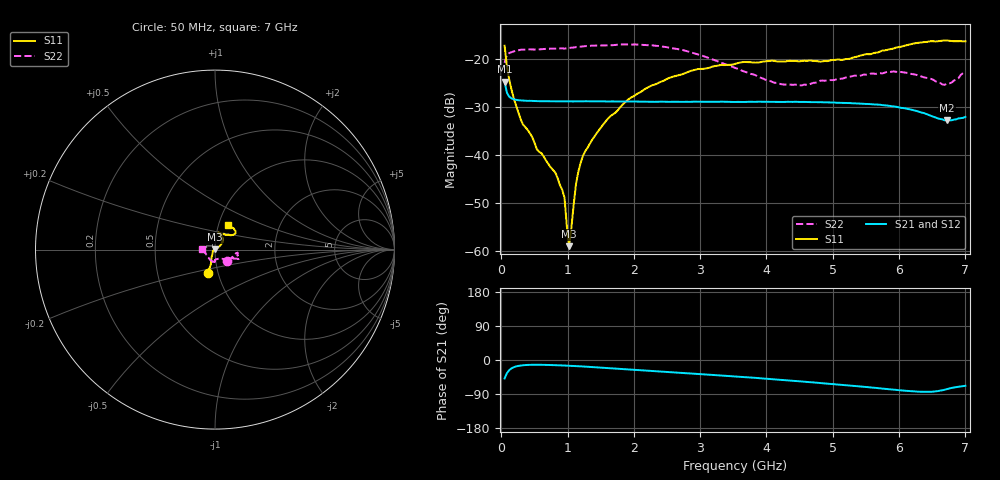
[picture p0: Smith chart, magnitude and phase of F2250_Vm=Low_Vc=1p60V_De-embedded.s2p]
! Integrated Device Technology
! Corporate Headquarters
! 6024 Silver Creek Valley Road
! San Jose, CA 95138  USA
! Phone:  1-408-284-8200
! Toll Free:  1-800-223-1366
! Webpage:  http://www.idt.com/
! Timing and RF Division
! 515 Groton Road, Suite 102
! Westford, MA 01886-6024
! Device:  F2250
! Description: Voltage Variable RF Attenuator
! Frequency:  50.0 -  6000.00 MHz
! Package:  3x3 mm Thin QFN Plastic Package: 16 pin
! Ports:  2 RF, 3 DC
!  Pin  1  = GND
!  Pin  2  = NC
!  Pin  3  = RF1  = Port 1
!  Pin  4  = NC
!  Pin  5  = GND
!  Pin  6  = GND
!  Pin  7  = GND
!  Pin  8  = GND
!  Pin  9  = NC
!  Pin 10  = RF2  = Port 2
!  Pin 11  = NC
!  Pin 12  = GND
!  Pin 13  = GND
!  Pin 14  = VCNTRL
!  Pin 15  = VDD
!  Pin 16  = VMODE
! Vcntrl:  1.600 Volts
! Vmode:  +0.000 Volts
! Vdd:  +3.30  Volts
! Current:  1.190 mA
! Data:  The device was measured on a the F2250 evaluation board which has
!  individual transmission lines to the RF pins.  Data was collected
!  using a calibrated network analyzer.  The evaluation board was
!  de-embedded using a TRL calibration technique.
!  The reference plane is the edge of the package pin.
! Misc:  SN 10
!  Action Tracker AT0258
! Date Measured:  2014-11-26
! Date:  2015-10-15  MJV
! Note:
!  Integrated Device Technology supplies this data as a sample of measured
!  data at the package pin for this product.  Your particular data for this
!  product may vary.
!  Data was taken at 25 degrees C.
!  Integrated Device Technology reserves the right to change this data at anytime.
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# GHz S dB R 50
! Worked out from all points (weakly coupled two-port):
!   201 points, 50 MHz to 7 GHz, reference 50 ohm
!   highest |S21| = -24.68 dB at 50 MHz (marker M1); lowest = -32.7 dB at 6.722 GHz (marker M2)
!   lowest |S11| = -59.0 dB at 1.023 GHz (marker M3), VSWR 1.00, Z = 50 + j0.103 ohm
!   |S11| at or under -10 dB: start of sweep to end of sweep
!   |S22| runs from -25.5 to -16.9 dB; largest |S21 - S12| = 0.00022
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0.05  -17.16 -107.3  -24.68 -48.7  -24.68 -48.7  -20.72 -41.6
0.1195  -24.26 -109.6  -27.81 -26.8  -27.79 -26.7  -18.69 -12.2
0.29325  -32.56 -122.7  -28.59 -14.6  -28.57 -14.6  -17.99 -8.4
0.467  -36.25 -141.3  -28.69 -12.6  -28.71 -12.6  -17.94 -8.0
0.5365  -38.79 -148.6  -28.74 -12.6  -28.74 -12.6  -17.94 -9.1
0.8145  -43.66 176.0  -28.77 -13.7  -28.79 -13.7  -17.76 -12.9
0.91875  -47.26 156.3  -28.79 -14.4  -28.81 -14.4  -17.70 -14.6
0.9535  -48.92 175.4  -28.80 -14.6  -28.81 -14.6  -17.77 -14.8
0.98825  -54.83 160.0  -28.80 -14.9  -28.82 -14.9  -17.68 -15.0
1.023  -59.04 112.1  -28.79 -15.2  -28.84 -15.1  -17.63 -15.0
1.12725  -46.02 38.8  -28.78 -16.1  -28.80 -16.1  -17.46 -16.4
1.2315  -40.14 31.9  -28.78 -17.1  -28.78 -17.1  -17.29 -17.8
1.6485  -31.85 37.2  -28.79 -21.6  -28.80 -21.6  -17.07 -20.0
1.9265  -28.26 38.2  -28.82 -24.7  -28.80 -24.7  -16.89 -21.2
2.37825  -24.86 45.1  -28.85 -29.8  -28.84 -29.9  -17.22 -22.6
2.93425  -22.12 58.5  -28.86 -36.3  -28.88 -36.3  -18.82 -25.5
3.525  -20.95 71.5  -28.92 -43.4  -28.91 -43.5  -21.78 -39.3
4.22  -20.44 77.8  -28.90 -52.2  -28.92 -52.2  -25.19 -66.9
4.7065  -20.35 71.8  -28.94 -59.2  -28.94 -59.2  -24.91 -86.9
5.85325  -17.91 39.8  -29.73 -77.2  -29.74 -77.3  -22.66 -92.6
6.722  -16.08 49.7  -32.75 -76.9  -32.77 -76.9  -25.08 -149.7
7  -16.23 62.8  -32.02 -68.0  -32.06 -67.9  -22.50 177.1
